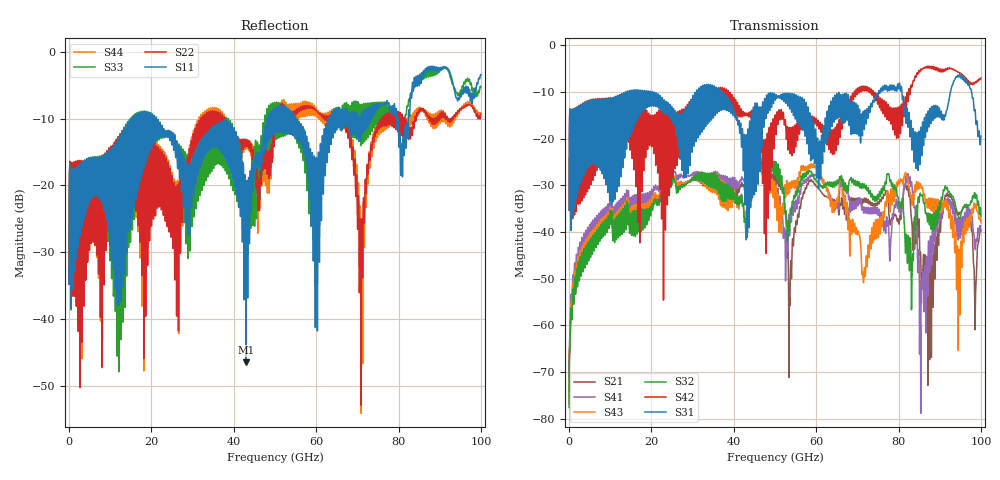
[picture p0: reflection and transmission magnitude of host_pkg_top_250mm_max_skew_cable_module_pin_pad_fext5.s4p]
# Hz S RI R 50
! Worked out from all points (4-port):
!   10000 points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, 10 MHz to 100 GHz, reference 50 ohm
!   strongest paths, dB at 10 MHz, 25.01 GHz, 50.01 GHz, 75.01 GHz, 100 GHz:
!     S31: -35.3, -14.2, -11.6, -10.7, -19.5
!     S42: -35.3, -14.4, -15.0, -11.9, -7.0
!     S32: -77.6, -29.5, -27.6, -32.1, -36.6
!     S43: -76.9, -28.7, -33.9, -39.7, -38.0
!     S41: -75.8, -27.8, -31.5, -35.9, -39.6
!     S21: -76.8, -29.5, -29.2, -33.5, -39.6
!   lowest |S11| = -46.5 dB at 42.95 GHz (marker M1), VSWR 1.01, Z = 49.5 - j0.0805 ohm
!   |S11| at or under -10 dB: start of sweep to 15.11 GHz; 21.17 GHz to 48.05 GHz (26.89 GHz wide, 77.7 % of centre); 55.02 GHz to 62.91 GHz (7.887 GHz wide, 13.4 % of centre)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
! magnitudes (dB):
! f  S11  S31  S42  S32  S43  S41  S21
! 10 MHz  -34.8  -35.3  -35.3  -77.6  -76.9  -75.8  -76.8
! 9.91 GHz  -24.2  -19.6  -17.0  -35.4  -34.7  -33.1  -34.6
! 42.95 GHz  -46.5  -19.4  -14.9  -41.6  -37.1  -30.4  -32.0
! 53.62 GHz  -8.8  -13.0  -22.4  -37.2  -30.1  -38.2  -55.4
! 70.88 GHz  -12.2  -16.9  -9.9  -29.9  -43.7  -33.2  -33.6
! 85.53 GHz  -3.6  -20.4  -5.3  -32.2  -30.5  -51.3  -54.9
! 100 GHz  -3.4  -19.5  -7.0  -36.6  -38.0  -39.6  -39.6
